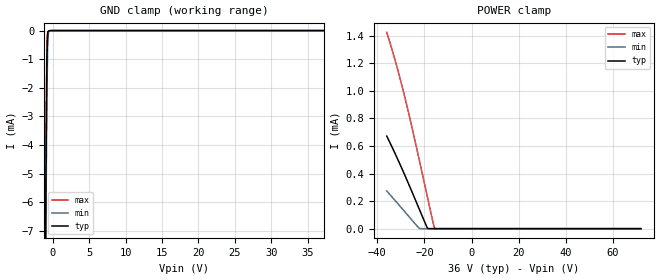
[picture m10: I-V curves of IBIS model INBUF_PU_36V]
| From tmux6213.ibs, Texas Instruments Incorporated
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| Model11
[Model]   INBUF_PU_36V
Model_type   Input
Vinl = 0.8
Vinh = 1.3
|   typ   min   max
C_comp   1.85pF   1.7pF   2.1pF
[Voltage Range]   36   32.4   39.6
[Temperature Range]   27   125   -40
[Power Clamp Reference]   36   32.4   39.6
[GND Clamp Reference]   0   0   0
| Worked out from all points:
|   GND clamp passes 1 mA (typ) near -0.80 V on its own axis
[GND Clamp]
|   Voltage   I(typ)   I(min)   I(max)
-36V      -1.895A    -1.893A    -1.898A
-1.008V   -8.362mA   -9.819mA   -7.209mA
-900mV    -3.84mA    -5.377mA   -2.655mA
-792mV    -816.2uA   -2.014mA   -233.9uA
-684mV    -54.17uA   -360uA     -43.74uA
-576mV    -14.96uA   -29.78uA   -22.95uA
-360mV    -930.3nA   -1.246uA   -1.146uA
72V       0A         0A         0A
[POWER Clamp]
|   Voltage   I(typ)   I(min)   I(max)
-36V      672.1uA    273.8uA    1.425mA
-32.54V   548.6uA    206.4uA    1.229mA
-28.98V   413.9uA    135.7uA    1mA
-25.85V   290.2uA    73.06uA    776.8uA
-22.07V   137uA      1.101uA    490uA
-18.72V   4.848uA    0A         229.5uA
-16.24V   0A         0A         38.21uA
-15.8V    0A         0A         8.402uA
-15.59V   0A         0A         340.8nA
72V       0A         0A         0A
